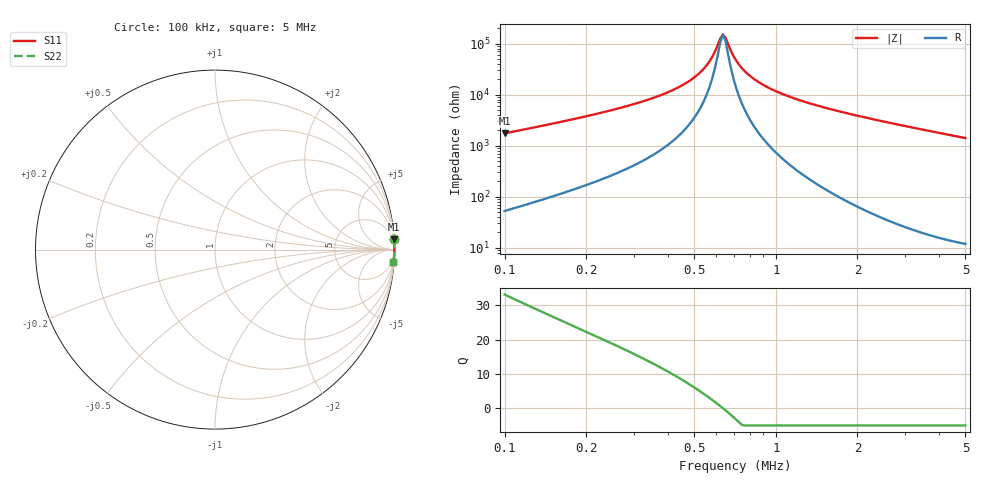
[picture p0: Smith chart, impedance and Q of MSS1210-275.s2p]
# MHz S MA R 50
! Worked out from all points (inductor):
!   172 points, 100 kHz to 5 MHz, reference 50 ohm
!   read as one part in series: L = 2.7 mH near 100 kHz
!   highest Q = 33.2 at 100 kHz (marker M1), where L = 2.77 mH
!   self-resonance near 637.9 kHz
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0.1  0.9966 3.3  0.05733 -85.0  0.05733 -85.0  0.9966 3.3
0.1377517  0.9977 2.3  0.04073 -85.6  0.04073 -85.6  0.9977 2.3
0.1854635  0.9983 1.7  0.02908 -85.9  0.02908 -85.9  0.9983 1.7
0.4130483  0.9991 0.5  0.008336 -83.9  0.008336 -83.9  0.9991 0.5
0.5074816  0.9992 0.2  0.004343 -79.9  0.004343 -79.9  0.9992 0.2
0.568981  0.9993 0.1  0.002249 -71.7  0.002249 -71.7  0.9993 0.1
0.5956193  0.9993 0.1  0.00146 -61.9  0.00146 -61.9  0.9993 0.1
0.6235048  0.9993 0.0  0.0008042 -33.5  0.0008042 -33.5  0.9993 0.0
0.6379333  0.9993 0.0  0.0006633 -1.9  0.0006633 -1.9  0.9993 0.0
0.6526957  0.9993 -0.0  0.000768 31.4  0.000768 31.4  0.9993 -0.0
0.6832533  0.9994 -0.1  0.0014 62.7  0.0014 62.7  0.9994 -0.1
0.6990645  0.9994 -0.1  0.001785 69.1  0.001785 69.1  0.9994 -0.1
0.7487274  0.9994 -0.2  0.003008 78.1  0.003008 78.1  0.9994 -0.2
0.8204757  0.9994 -0.3  0.004706 82.6  0.004706 82.6  0.9994 -0.3
0.9199055  0.9994 -0.4  0.006904 85.0  0.006904 85.0  0.9994 -0.4
1.055252  0.9994 -0.6  0.009672 86.3  0.009672 86.3  0.9994 -0.6
1.238525  0.9994 -0.8  0.01314 87.1  0.01314 87.1  0.9994 -0.8
1.745569  0.9993 -1.3  0.02184 87.6  0.02184 87.6  0.9993 -1.3
2.575376  0.999 -2.0  0.03489 87.3  0.03489 87.3  0.999 -2.0
3.388961  0.9984 -2.7  0.04716 86.7  0.04716 86.7  0.9984 -2.7
4.260117  0.9977 -3.4  0.06004 86.1  0.06004 86.1  0.9977 -3.4
5  0.9969 -4.1  0.07086 85.5  0.07086 85.5  0.9969 -4.1
